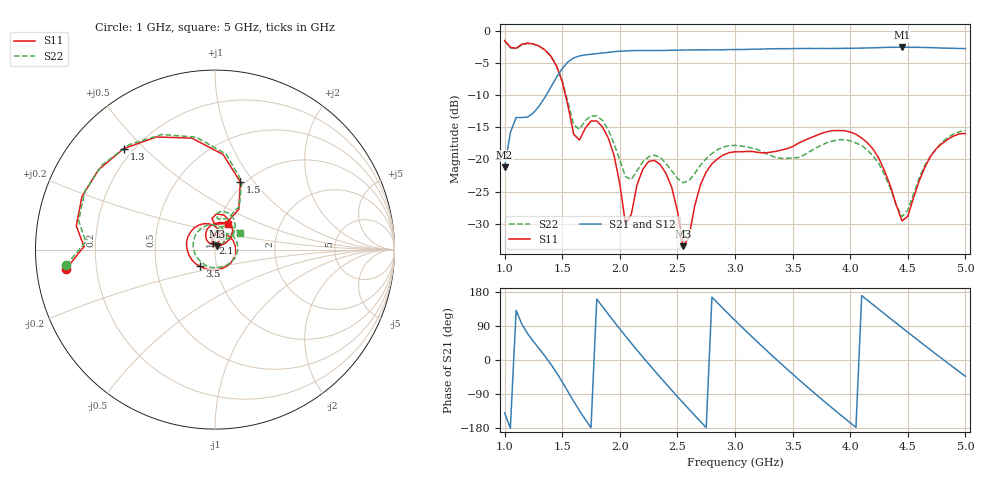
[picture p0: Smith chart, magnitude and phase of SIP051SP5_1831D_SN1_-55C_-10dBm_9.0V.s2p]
# GHz  S  dB  R  50
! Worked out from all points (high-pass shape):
!   81 points, 1 GHz to 5 GHz, reference 50 ohm
!   highest |S21| = -2.59 dB at 4.45 GHz (marker M1); lowest = -21.2 dB at 1 GHz (marker M2)
!   |S21| within 3 dB of the highest: 1.515 GHz to end of sweep
!   lowest |S11| = -33.5 dB at 2.55 GHz (marker M3), VSWR 1.04, Z = 51.2 + j1.81 ohm
!   |S11| at or under -10 dB: 1.528 GHz to end of sweep
!   |S22| runs from -28.9 to -1.6 dB; largest |S21 - S12| = 0.0025
!   S11 on the Smith chart (normalised r, x): 1 GHz: 0.09, -0.07; 1.3 GHz: 0.16, +0.43; 1.5 GHz: 0.95, +0.86; 2.1 GHz: 0.98, +0.07; 3.5 GHz: 0.83, -0.15; 5 GHz: 1.11, +0.32
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1  -1.53 -172.5  -21.24 -139.6  -21.24 -139.6  -1.57 -174.1
1.1  -2.74 178.8  -13.50 130.8  -13.49 130.8  -2.84 176.6
1.3  -2.40 132.1  -11.70 29.8  -11.71 29.9  -2.43 129.3
1.5  -7.92 69.4  -5.90 -57.7  -5.89 -57.7  -7.74 68.8
1.6  -16.09 67.1  -4.25 -109.1  -4.24 -109.2  -14.66 68.1
1.7  -15.15 95.5  -3.78 -156.6  -3.78 -156.7  -13.98 87.6
1.9  -16.68 47.6  -3.39 120.9  -3.37 121.0  -15.39 48.0
2.05  -30.05 53.8  -3.16 63.0  -3.17 63.0  -22.70 48.3
2.1  -28.50 105.9  -3.12 44.1  -3.12 44.3  -23.12 65.7
2.2  -21.51 99.9  -3.10 7.6  -3.10 7.6  -20.37 72.9
2.35  -20.78 61.2  -3.09 -45.3  -3.09 -45.2  -19.68 53.1
2.55  -33.47 56.3  -3.02 -113.1  -3.02 -113.2  -23.62 51.4
2.75  -21.95 88.8  -3.00 -178.4  -3.00 -178.3  -19.87 59.4
3  -18.82 10.2  -2.95 104.7  -2.95 104.6  -17.82 18.0
3.3  -18.90 -84.4  -2.84 17.8  -2.85 17.8  -19.32 -52.5
3.5  -18.02 -133.4  -2.80 -37.1  -2.80 -37.2  -19.78 -118.3
3.7  -16.32 -175.7  -2.78 -90.0  -2.78 -90.0  -18.25 173.6
4.05  -16.09 112.8  -2.74 -177.8  -2.74 -177.9  -17.45 84.8
4.35  -24.18 64.9  -2.60 109.3  -2.62 109.3  -24.56 38.7
4.45  -29.56 87.5  -2.59 85.2  -2.58 85.3  -28.90 63.8
4.75  -18.29 110.9  -2.68 14.3  -2.69 14.3  -18.28 79.7
5  -15.98 61.9  -2.79 -42.9  -2.80 -43.0  -15.52 34.5
